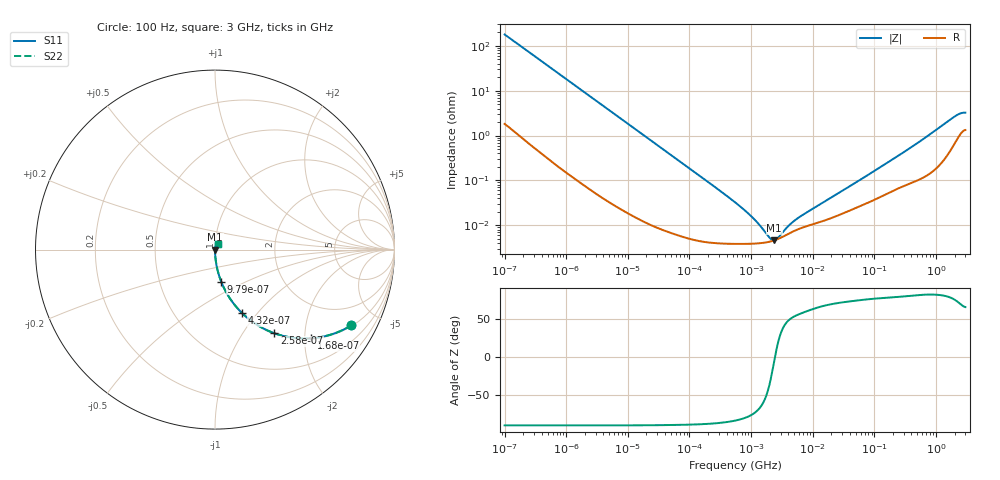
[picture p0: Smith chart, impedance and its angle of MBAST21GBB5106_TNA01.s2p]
! MBAST21GBB5106_TNA01  S-PARAMETER MODEL  ( Standard Model )
! Model Generated by TAIYO YUDEN Corporation (http://www.ty-top.com)
! Version 2.0
! TAIYO YUDEN Control No. 231201
! Copyright(c) 2014 TAIYO YUDEN CO.,LTD. All Rights Reserved.
! Product Description (link to TY-COMPAS)
! https://ds.yuden.co.jp/TYCOMPAS/or/detail?pn=MBAST21GBB5106KTNA01&u=M
! Products Name : Multilayer Ceramic Capacitors
! Characteristics :
!  Capacitance : 10 [uF] , Rated Voltage : 25 [V] , TCC : X5R
!  Case Size : 2.0 x 1.25 / 0.079 x 0.049 [mm/inch] , Thickness : 1.25 / 0.049 [mm/inch]
!  (Conditions: Temperature = 25 [degC] , DC Bias Voltage = 0 [V])
! External Node Assignments :
!  1  o---| |---o  2
! GND o---------o GND
! Frequency Range : 100Hz  -  3GHz  [ 401 STEP ]
# MHZ S RI R 50
! Freq[MHz].  S11 Real  S11 Imag  S21 Real  S21 Imag  S12 Real  S12 Imag  S22 Real  S22 Imag
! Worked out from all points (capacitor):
!   401 points, 100 Hz to 3 GHz, reference 50 ohm
!   read as one part in series: C = 8.87 uF near 109 Hz
!   lowest |Z| = 4.62 mohm at 2.367 MHz (marker M1)
!   series resonance near 2.435 MHz, so ESL is about 480 pH
!   S11 on the Smith chart (normalised r, x): 100 Hz: 1.04, -3.58; 168 Hz: 1.02, -2.15; 258 Hz: 1.01, -1.40; 432 Hz: 1.01, -0.84; 979 Hz: 1.00, -0.37; 3 GHz: 1.03, +0.06
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0.0001  0.7601 -0.422  0.2399 0.422  0.2399 0.422  0.7601 -0.422
0.000119  0.6933 -0.4561  0.3067 0.4561  0.3067 0.4561  0.6933 -0.4561
0.000168  0.5347 -0.494  0.4653 0.494  0.4653 0.494  0.5347 -0.494
0.000258  0.3299 -0.4657  0.6701 0.4657  0.6701 0.4657  0.3299 -0.4657
0.000432  0.1511 -0.3539  0.8489 0.3539  0.8489 0.3539  0.1511 -0.3539
0.000636  0.0768 -0.2621  0.9232 0.2621  0.9232 0.2621  0.0768 -0.2621
0.000979  0.0346 -0.1787  0.9654 0.1787  0.9654 0.1787  0.0346 -0.1787
0.001788  0.0111 -0.1006  0.9889 0.1006  0.9889 0.1006  0.0111 -0.1006
0.005476  0.00141 -0.0334  0.9986 0.0334  0.9986 0.0334  0.00141 -0.0334
0.031977  0.000118 -0.00577  0.9999 0.00577  0.9999 0.00577  0.000118 -0.00577
0.547723  3.86e-05 -0.000324  1 0.000324  1 0.000324  3.86e-05 -0.000324
0.87939  3.86e-05 -0.000185  1 0.000185  1 0.000185  3.86e-05 -0.000185
1.352413  3.97e-05 -9.55e-05  1 9.55e-05  1 9.55e-05  3.97e-05 -9.55e-05
1.53882  4.05e-05 -7.28e-05  1 7.28e-05  1 7.28e-05  4.05e-05 -7.28e-05
2.366551  4.6e-05 -4.28e-06  1 4.28e-06  1 4.28e-06  4.6e-05 -4.28e-06
4.141163  6.57e-05 7.58e-05  0.9999 -7.58e-05  0.9999 -7.58e-05  6.57e-05 7.58e-05
9.794414  0.000104 0.000204  0.9999 -0.000204  0.9999 -0.000204  0.000104 0.000204
175.1444  0.000543 0.0026  0.9995 -0.0026  0.9995 -0.0026  0.000543 0.0026
513.708  0.00106 0.00688  0.9989 -0.00688  0.9989 -0.00688  0.00106 0.00688
1950.712  0.00678 0.0248  0.9932 -0.0248  0.9932 -0.0248  0.00678 0.0248
2419.119  0.0109 0.0283  0.9891 -0.0283  0.9891 -0.0283  0.0109 0.0283
3000  0.0139 0.0288  0.9861 -0.0288  0.9861 -0.0288  0.0139 0.0288
